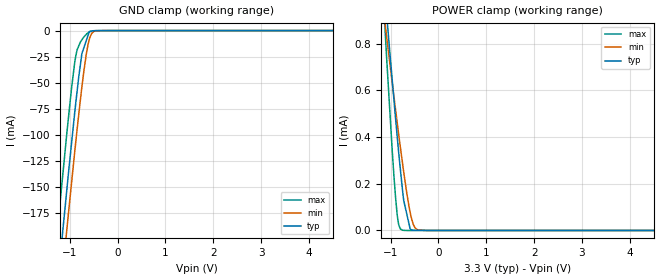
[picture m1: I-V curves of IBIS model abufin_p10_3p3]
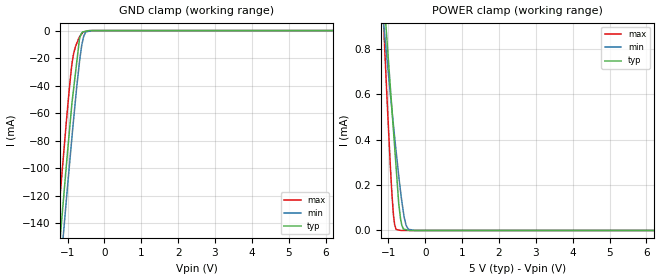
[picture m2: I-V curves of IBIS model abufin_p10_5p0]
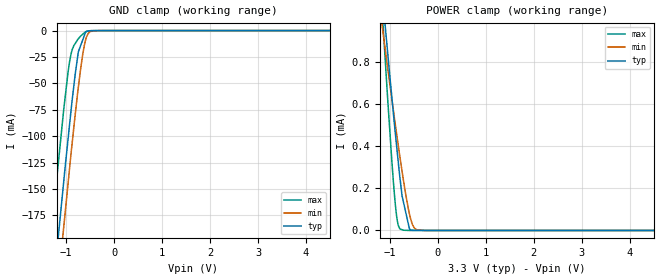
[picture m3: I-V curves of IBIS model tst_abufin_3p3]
|Texas Instruments Incorporated
| 24-Channel, 12-Bit PWM LED Driver with Internal Oscillator
| Marketing part#   Digital Voltage Range   Package-type   #pins
| TLC5947DAP   3.0-5.5V   HTSSOP   32
| TLC5947DAPG4   3.0-5.5V   HTSSOP   32
| TLC5947DAPR   3.0-5.5V   HTSSOP   32
| TLC5947DAPRG4   3.0-5.5V   HTSSOP   32
| TLC5947RHBR   3.0-5.5V   QFN   32
| TLC5947RHBRG4   3.0-5.5V   QFN   32
| TLC5947RHBT   3.0-5.5V   QFN   32
| TLC5947RHBTG4   3.0-5.5V   QFN   32
[IBIS Ver]   3.2
[File name]   tlc5947.ibs
|SIMDE Ver   V2.2 - 201009 - RHL4 - Build 420
[File Rev]   1.0
[Date]   10/19/2010
[Source]
| Texas Instruments Incorporated.
| Analog-eLab Design Center, HPA
| 12500 TI Blvd
| Dallas, TX -75243
| e-mail: elab_ibis@list.ti.com
| -Model generated from simulations in TISPICE
[Notes]   Revision History:
| Rev 1.0: 10/19/2010
| - Initial version of the model
| - Model generated from simulations in TISPICE
| - Model matched to SPICE simulation
| - C_comp although listed in numerical order of value are
|   obtained from varying PVT conditions. For PVT conditions for
|   each specific value refer the buffer description under
|   respective [Model]. IBIS model user is responsible for using
|   appropriate C_comp to simulate for Signal Integrity.
[Disclaimer]
| This model is designed as an aid for customers of Texas Instruments.
| TI and its licensors and suppliers make no warranties, either expressed
| or implied, with respect to this  model, including the warranties of
| merchantability or fitness for a particular purpose. The model is
| provided solely on an "as is" basis. The entire risk as to its quality
| and performance is with the customer.
[Copyright]
 (C) Copyright 2010 Texas Instruments Incorporated.All rights reserved.
|   TLC5947
[Component]   TLC5947DAP-HTSSOP
[Manufacturer]   TI
[Package]   |32 HTTSOP - DAP package
|   typ   min   max
R_pkg   0.11963   0.09598   0.14689
L_pkg   3.10801nH   2.51317nH   3.94310nH
C_pkg   0.49824pF   0.38041pF   0.69822pF
[Pin]  signal_name   model_name   R_pin   L_pin   C_pin
1   GND   GND   0.04251   3.43118nH  0.76378pF
2   BLANK   TST_ABUFIN   0.09598   3.37800nH  0.66748pF
3   SCLK   ABUFIN_P10   0.10699   3.18227nH  0.59525pF
4   SIN   ABUFIN_P10   0.13166   3.30824nH  0.51461pF
5   OUT0   TERM   0.14689   3.20355nH  0.41796pF
6   OUT1   TERM   0.13031   2.90412nH  0.40400pF
7   OUT2   TERM   0.11837   2.66352nH  0.39029pF
8   OUT3   TERM   0.11081   2.52898nH  0.38148pF
9   OUT4   TERM   0.10985   2.51317nH  0.38043pF
10   OUT5   TERM   0.11565   2.61843nH  0.38732pF
11   OUT6   TERM   0.12633   2.83818nH  0.39953pF
12   OUT7   TERM   0.14196   3.12171nH  0.41379pF
13   OUT8   TERM   0.12900   3.34240nH  0.51749pF
14   OUT9   TERM   0.11666   3.41551nH  0.62621pF
15   OUT10   TERM   0.10582   3.60496nH  0.68361pF
16   OUT11   TERM   0.09811   3.94310nH  0.69822pF
17   OUT12   TERM   0.09770   3.84908nH  0.68749pF
18   OUT13   TERM   0.10545   3.55492nH  0.67834pF
19   OUT14   TERM   0.11649   3.36112nH  0.60674pF
20   OUT15   TERM   0.13095   3.30561nH  0.51740pF
21   OUT16   TERM   0.14196   3.12197nH  0.41467pF
22   OUT17   TERM   0.12633   2.83833nH  0.39949pF
23   OUT18   TERM   0.11565   2.61862nH  0.38725pF
24   OUT19   TERM   0.10985   2.51324nH  0.38041pF
25   OUT20   TERM   0.11081   2.52904nH  0.38148pF
26   OUT21   TERM   0.11837   2.66352nH  0.39032pF
27   OUT22   TERM   0.13031   2.90413nH  0.40412pF
28   OUT23   TERM   0.14688   3.20329nH  0.41946pF
29   SOUT   SOUTBUF   0.13543   3.37689nH  0.52246pF
30   XLAT   ABUFIN_P10   0.11543   3.33356nH  0.60637pF
31   IREF   TERM   0.10287   3.50082nH  0.67349pF
32   VCC   POWER   0.09952   3.87316nH  0.68748pF
|   TLC5947
[Component]   TLC5947RHB-QFN
[Manufacturer]   TI
[Package]   |32 QFN - RHB package
|   typ   min   max
R_pkg   0.08200   0.03662   0.11120
L_pkg   1.41989nH   0.68193nH   1.93473nH
C_pkg   0.20552pF   0.16635pF   0.28093pF
[Pin]  signal_name   model_name   R_pin   L_pin   C_pin
1   OUT0   TERM   0.04346   0.80188nH  0.28093pF
2   OUT1   TERM   0.10001   1.72968nH  0.20792pF
3   OUT2   TERM   0.04181   0.76954nH  0.26970pF
4   OUT3   TERM   0.08712   1.49358nH  0.19139pF
5   OUT4   TERM   0.08627   1.47818nH  0.19032pF
6   OUT5   TERM   0.08951   1.53727nH  0.19445pF
7   OUT6   TERM   0.09636   1.66279nH  0.20329pF
8   OUT7   TERM   0.10667   1.85843nH  0.19785pF
9   OUT8   TERM   0.10191   1.76992nH  0.18993pF
10   OUT9   TERM   0.00074   0.14328nH  0.10231pF
11   OUT10   TERM   0.00074   0.14227nH  0.10237pF
12   OUT11   TERM   0.06770   1.13926nH  0.16635pF
13   OUT12   TERM   0.06775   1.14379nH  0.16649pF
14   OUT13   TERM   0.08434   1.43739nH  0.18658pF
15   OUT14   TERM   0.07240   1.22550nH  0.17408pF
16   OUT15   TERM   0.10191   1.76483nH  0.18989pF
17   OUT16   TERM   0.10667   1.85112nH  0.19766pF
18   OUT17   TERM   0.04170   0.76742nH  0.27259pF
19   OUT18   TERM   0.04371   0.79955nH  0.27598pF
20   OUT19   TERM   0.08627   1.46918nH  0.19005pF
21   OUT20   TERM   0.08712   1.48469nH  0.19112pF
22   OUT21   TERM   0.09193   1.57278nH  0.19727pF
23   OUT22   TERM   0.10001   1.72209nH  0.20782pF
24   OUT23   TERM   0.11120   1.93473nH  0.20255pF
25   SOUT   SOUTBUF   0.10602   1.84052nH  0.19353pF
26   XLAT   ABUFIN_P10   0.00074   0.14328nH  0.10231pF
27   IREF   TERM   0.00074   0.14227nH  0.10237pF
28   VCC   POWER   0.06753   1.13951nH  0.16621pF
29   GND   GND   0.06217   1.04518nH  0.16421pF
30   BLANK   TST_ABUFIN   0.03662   0.68193nH  0.24624pF
31   SCLK   ABUFIN_P10   0.07093   1.19898nH  0.17131pF
32   SIN   ABUFIN_P10   0.10258   1.78210nH  0.18810pF
33   thermal_pad   NC   0.00067   0.24694nH  2.29047pF
|   Model Selectors
[Model Selector] ABUFIN_P10
abufin_p10_3p3   3.3V digital input
abufin_p10_5p0   5.0V digital input
[Model Selector] SOUTBUF
soutbuf_3p3   3.3V digital Output
soutbuf_5p0   5.0V digital Output
[Model Selector] TST_ABUFIN
tst_abufin_3p3   3.3V digital Input
tst_abufin_5p0   5.0V digital Input
[Model Selector] TERM
TERM_3p3  3.3V nominal termination
TERM_5p0  5.0V nominal termination
|   Terminator Models
[Model]  TERM_3p3
Model_type Terminator
C_comp   1.0e-20F  1.0e-20F  1.0e-20F
|   typ   min   max
[Voltage Range]   3.3V   3.0V   3.6V
[POWER Clamp Reference]   3.3V   3.0V   3.6V
[GND Clamp Reference]   0V   0V   0V
|Ambient Temperature   65   125   -40
|Junction Temperature
[Temperature Range]   65   125   -40
[Model]  TERM_5p0
Model_type Terminator
C_comp   1.0e-20F  1.0e-20F  1.0e-20F
|   typ   min   max
[Voltage Range]   5.0V   4.5V   5.5V
[POWER Clamp Reference]   5.0V   4.5V   5.5V
[GND Clamp Reference]   0V   0V   0V
|Ambient Temperature   65   125   -40
|Junction Temperature
[Temperature Range]   65   125   -40
| Models and submodels in the file (8): abufin_p10_3p3 (Input), abufin_p10_5p0 (Input), tst_abufin_3p3 (Input), tst_abufin_5p0 (Input), soutbuf_3p3 (Output), soutbuf_5p0 (Output), TERM_3p3 (Terminator), TERM_5p0 (Terminator)
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|   abufin_p10_3p3 Model
[Model]   abufin_p10_3p3
Model_type   Input
Vinl = 0.99
Vinh = 2.31
|   typ   min   max
|   (nom PVT)   (Fast PVT)   (slow PVT)
|Average
C_comp   1.244e-12   1.242e-12   1.262e-12
| Where nom  PVT is Nominal Process,  3.3V,  65C
|   Fast PVT is Strong Process,   3.6V,  -40C
|   Slow PVT is Weak Process,   3V,  125C
[Model Spec]
|   typ   min   max
Vinl   0.99   0.9   1.08
Vinh   2.31   2.1   2.52
[Voltage Range]   3.3   3   3.6
|Ambient Temperature   25   85   -40
|Junction Temperature
[Temperature Range]   65   125   -40
[Power Clamp Reference]   3.3   3   3.6
[GND Clamp Reference]   0   0   0
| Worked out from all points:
|   GND clamp passes 1 mA (typ) near -0.59 V on its own axis
|   POWER clamp passes 1 mA (typ) near -1.11 V on its own axis
[GND Clamp]
|   Voltage   I(typ)   I(min)   I(max)
-3V       -1.103A    -1.135A    -1.06A
-1.369V   -298.7mA   -337.1mA   -246.4mA
-1.217V   -225.8mA   -264mA     -172.1mA
-1.168V   -202.7mA   -240.9mA   -149.2mA
-1.062V   -153.3mA   -191.4mA   -99.17mA
-964.8mV  -109.3mA   -147.3mA   -56.38mA
-871.2mV  -68.33mA   -105.7mA   -23.74mA
-745.8mV  -22mA      -54.17mA   -8.826mA
-590.7mV  -1.03mA    -8.343mA   -1.408mA
-495mV    -112.1uA   -826.6uA   -162.4uA
-321mV    -72.41uA   -5.947uA   -14.37uA
6V        0A         0A         0A
[POWER Clamp]
|   Voltage   I(typ)   I(min)   I(max)
-3V       5.884mA    4.247mA    8.074mA
-1.181V   1.169mA    999.4uA    1.098mA
-1.084V   928.3uA    831.4uA    742.5uA
-1.023V   779.1uA    728.4uA    535.8uA
-932.4mV  564.9uA    577.1uA    240.1uA
-864mV    407.6uA    464.8uA    71.07uA
-828mV    327.6uA    407uA      23.09uA
-741.6mV  155.7uA    274uA      617nA
-590.7mV  6.052uA    76.61uA    2.646nA
-528mV    757.2nA    27.04uA    1.59nA
-441mV    631.7nA    3.132uA    125.7pA
6V        0A         0A         0A
|   abufin_p10_5p0 Model
[Model]   abufin_p10_5p0
Model_type   Input
Vinl = 3.5
Vinh = 1.5
|   typ   min   max
|   (nom PVT)   (Fast PVT)   (slow PVT)
|Average
C_comp   1.178e-12   1.162e-12   1.277e-12
| Where nom  PVT is Nominal Process,  5V,  65C
|   Fast PVT is Strong Process,   5.5V,  -40C
|   Slow PVT is Weak Process,   4.5V,  125C
[Model Spec]
|   typ   min   max
Vinl   1.5   1.35   1.65
Vinh   3.5   3.15   3.85
[Voltage Range]   5   4.5   5.5
|Ambient Temperature   25   85   -40
|Junction Temperature
[Temperature Range]   65   125   -40
[Power Clamp Reference]   5   4.5   5.5
[GND Clamp Reference]   0   0   0
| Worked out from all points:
|   GND clamp passes 1 mA (typ) near -0.58 V on its own axis
|   POWER clamp passes 1 mA (typ) near -1.11 V on its own axis
[GND Clamp]
|   Voltage   I(typ)   I(min)   I(max)
-5V       -1.413A    -1.428A    -1.401A
-1.368V   -204.8mA   -228.9mA   -174.5mA
-1.183V   -145.4mA   -170mA     -113.9mA
-1.14V    -131.8mA   -156.7mA   -100.4mA
-1.045V   -102.1mA   -127.1mA   -70.25mA
-874.5mV  -51.37mA   -75.82mA   -23.19mA
-786.5mV  -31.35mA   -50.99mA   -11.8mA
-675mV    -5.992mA   -22.53mA   -4.604mA
-595mV    -1.123mA   -8.226mA   -1.565mA
-504mV    -498.3uA   -1.028mA   -604.3uA
-315mV    -805.2nA   -5.001uA   -3.36uA
10V       0A         0A         0A
[POWER Clamp]
|   Voltage   I(typ)   I(min)   I(max)
-5V       11.15mA    7.877mA    15.87mA
-1.14V    1.066mA    928.1uA    945.8uA
-1.111V   1.001mA    878.9uA    840.1uA
-1.023V   802.2uA    729.4uA    531.6uA
-902mV    529.3uA    527.5uA    155.9uA
-858mV    430.1uA    455.9uA    60.62uA
-786.5mV  268.8uA    342.1uA    4.269uA
-720mV    118.9uA    241.6uA    2.127uA
-665mV    46.09uA    165uA      354.9nA
-571.5mV  5.217uA    58.41uA    14.57nA
-459mV    944nA      5.127uA    11.73nA
10V       0A         0A         0A
|   tst_abufin_3p3 Model
[Model]   tst_abufin_3p3
Model_type   Input
Vinl = 0.99
Vinh = 2.31
|   typ   min   max
|   (nom PVT)   (Fast PVT)   (slow PVT)
|Average
C_comp   1.340e-12   1.330e-12   1.374e-12
| Where nom  PVT is Nominal Process,  3.3V,  65C
|   Fast PVT is Strong Process,   3.6V,  -40C
|   Slow PVT is Weak Process,   3V,  125C
[Model Spec]
|   typ   min   max
Vinl   0.99   0.9   1.08
Vinh   2.31   2.1   2.52
[Voltage Range]   3.3   3   3.6
|Ambient Temperature   25   85   -40
|Junction Temperature
[Temperature Range]   65   125   -40
[Power Clamp Reference]   3.3   3   3.6
[GND Clamp Reference]   0   0   0
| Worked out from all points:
|   GND clamp passes 1 mA (typ) near -0.59 V on its own axis
|   POWER clamp passes 1 mA (typ) near -1.11 V on its own axis
[GND Clamp]
|   Voltage   I(typ)   I(min)   I(max)
-3.3V     -1.244A    -1.282A    -1.18A
-1.382V   -299.2mA   -341.7mA   -229.1mA
-1.168V   -197.5mA   -240.3mA   -128mA
-1.051V   -143.6mA   -186.8mA   -75.43mA
-961.2mV  -103.5mA   -145.7mA   -39.96mA
-896.4mV  -75.22mA   -116.1mA   -21.92mA
-745.8mV  -20.23mA   -53.85mA   -7.804mA
-657mV    -9.22mA    -23.48mA   -3.593mA
-590.7mV  -1.002mA   -8.3mA     -1.277mA
-495mV    -111.7uA   -826.4uA   -138.3uA
-321mV    -72.15uA   -5.958uA   -14.35uA
6.6V      0A         0A         0A
[POWER Clamp]
|   Voltage   I(typ)   I(min)   I(max)
-3.3V     6.736mA    4.841mA    9.311mA
-1.146V   1.093mA    944uA      988uA
-1.122V   1.032mA    902.2uA    900.9uA
-1.044V   838.7uA    767.6uA    617.8uA
-954mV    620.4uA    614.8uA    314.5uA
-878.4mV  443.3uA    489.6uA    105.3uA
-824.4mV  323uA      402.1uA    23.76uA
-723.6mV  141.4uA    247.4uA    1.324uA
-590.7mV  6.156uA    76.64uA    105.7nA
-528mV    792.5nA    27.06uA    62.68nA
-444mV    665.6nA    3.407uA    5.077nA
6.6V      0A         0A         0A
